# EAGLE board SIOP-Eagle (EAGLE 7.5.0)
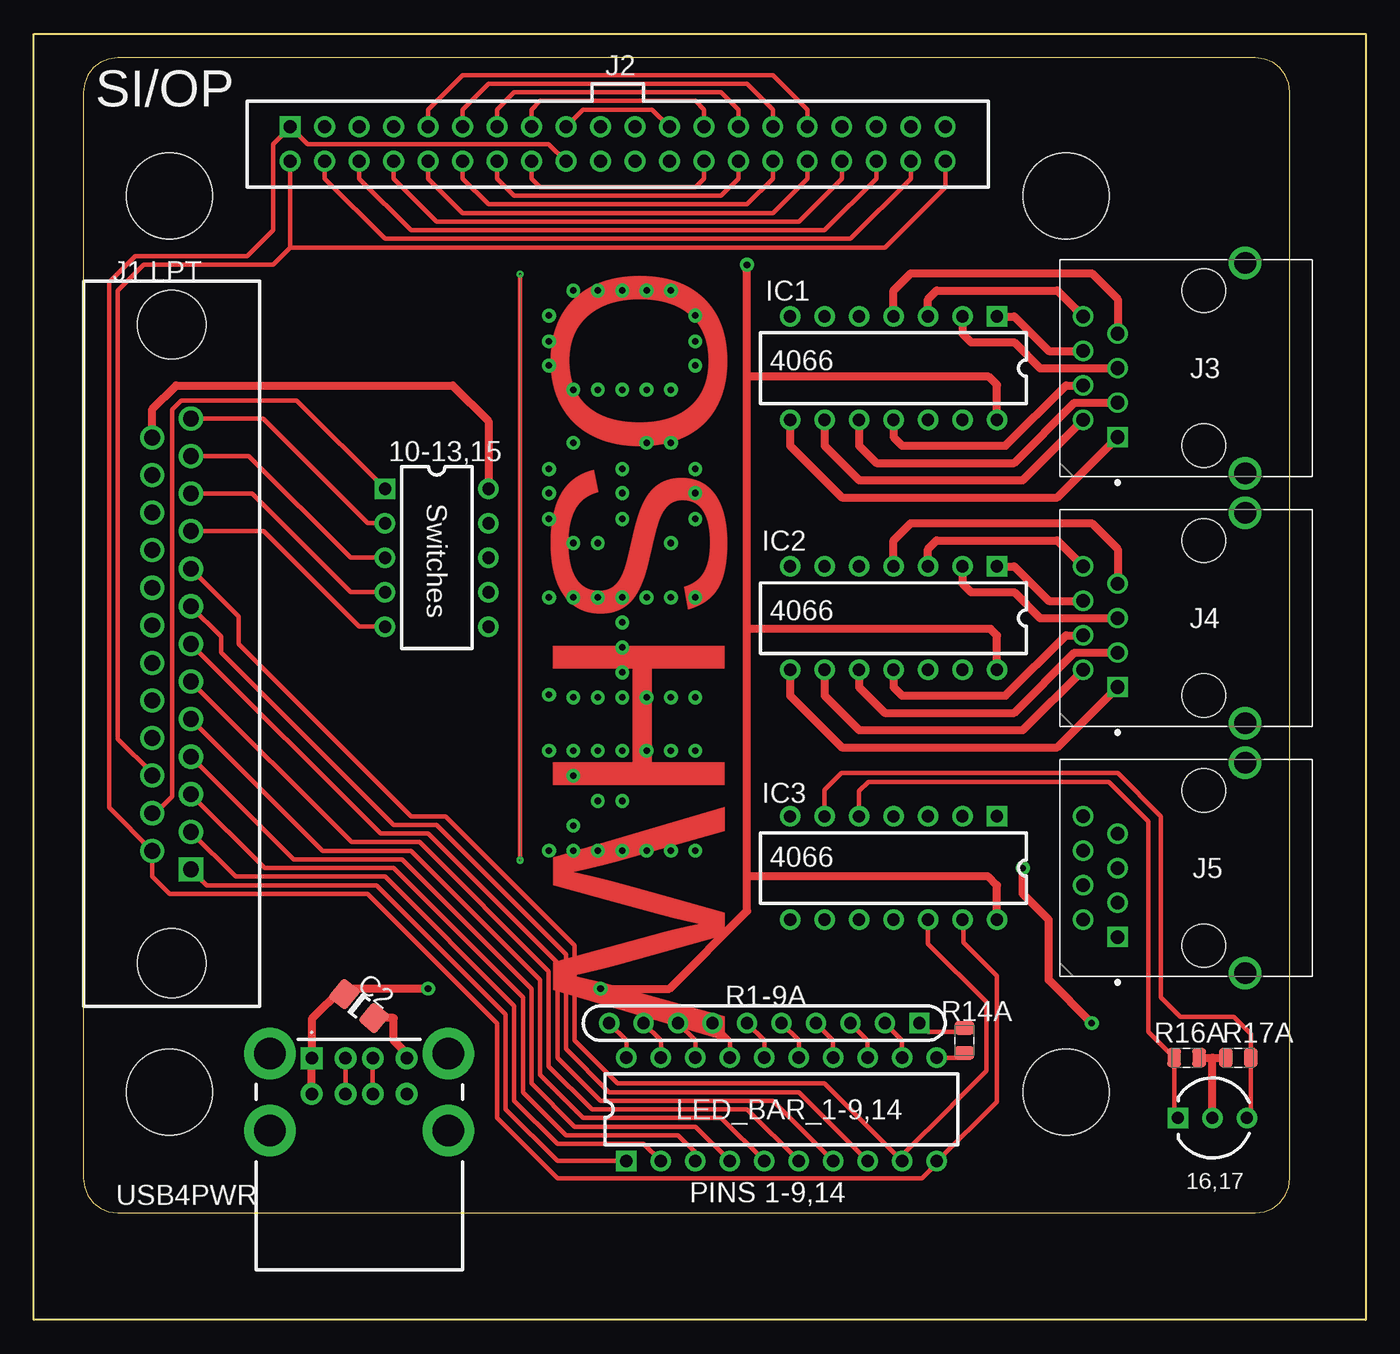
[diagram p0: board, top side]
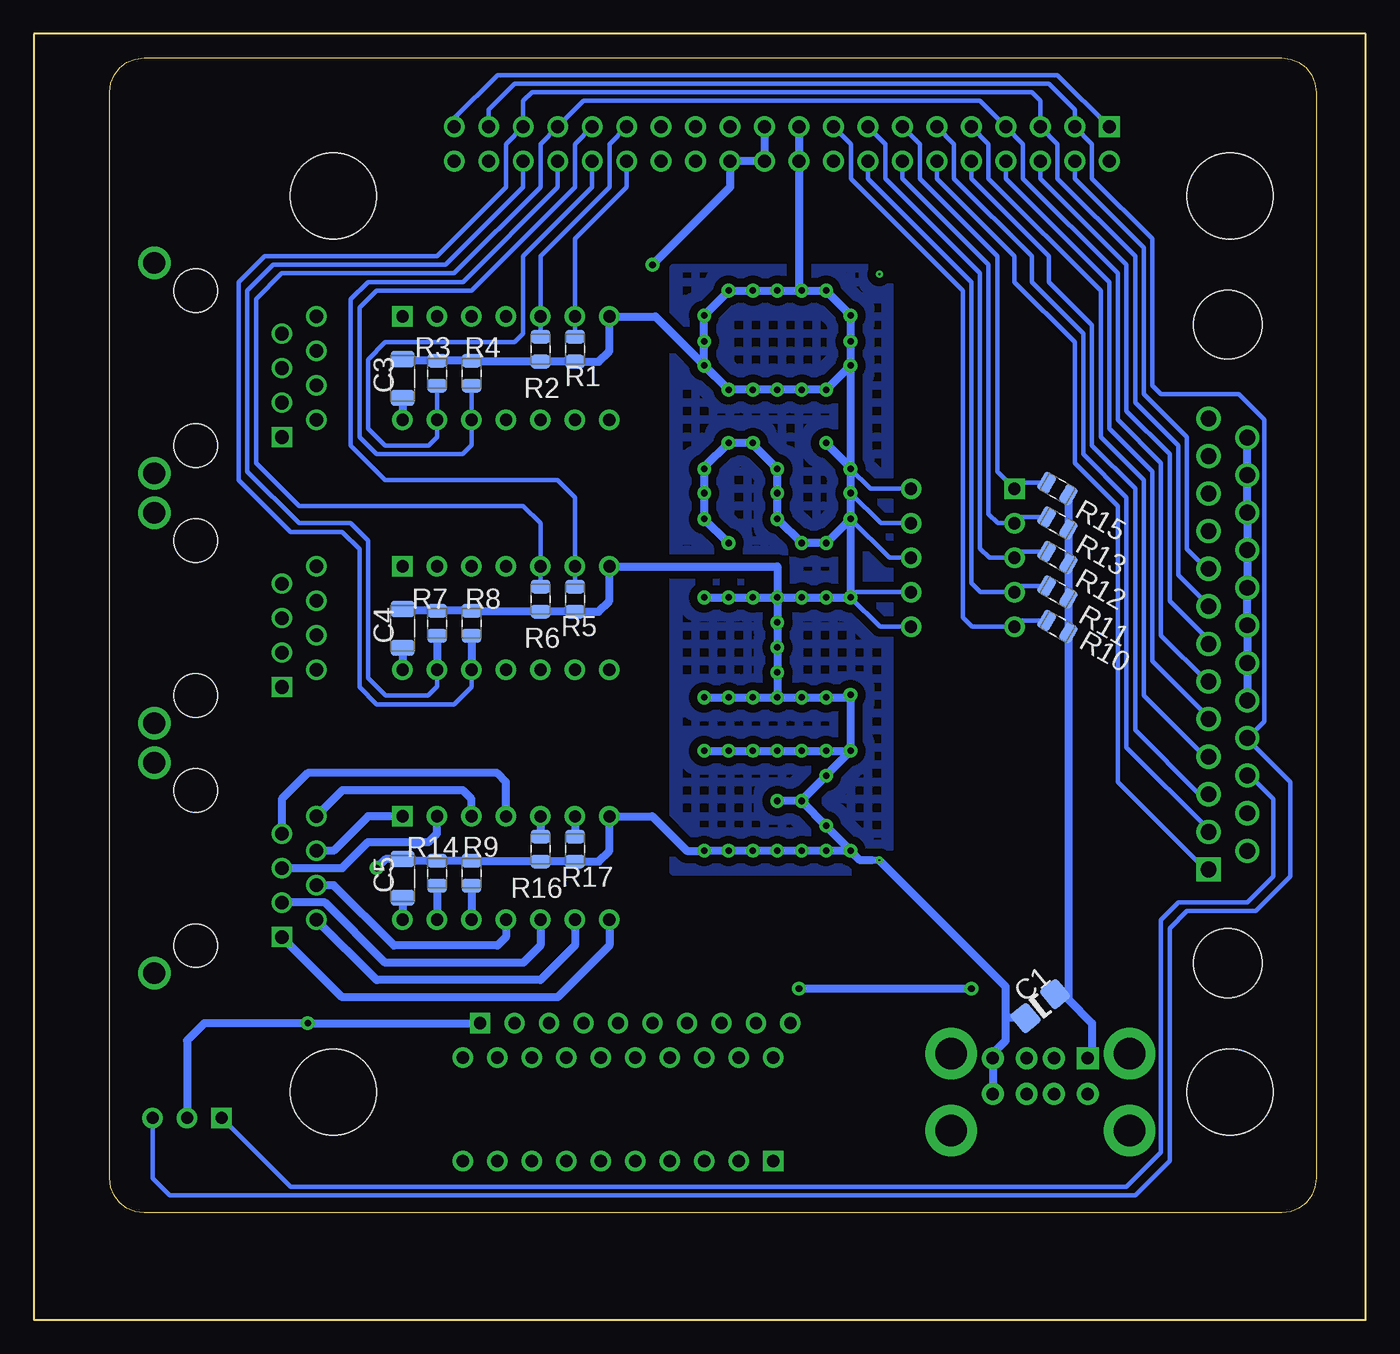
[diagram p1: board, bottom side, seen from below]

Size 98.11 x 94.73 mm. Coordinates in mm from the lower left corner, seen from the top.
Outline: 0,94.73 98.11,94.73 98.11,0 0,0 0,94.73
Copper layers (1*16): Top 0.035mm / dielectric 1.5mm / Bottom 0.035mm
Design rules "default *": minimum track width 10mil, minimum drill 0.61mm, track to track 8mil, track to pad 8mil, pad to pad 8mil, via to via 8mil, smd to smd 8mil, copper to edge 40mil, drill to drill 8mil, minimum pad ring 0mil, minimum via ring 8mil, stop-mask expansion 4mil, vias tented up to drill 40mil, thermal gap 10mil
Net classes: 0 Default: width 0.317 mm, clearance 0.597 mm
Holes 6.35 mm at 9.99,82.81 76.03,82.81 9.99,16.77 76.03,16.77
Milling: 28 lines

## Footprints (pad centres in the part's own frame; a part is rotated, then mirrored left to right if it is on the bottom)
CAP_1206 = smd 1.6 x 1.8: 1 -1.4,0; 2 1.4,0
CAP_1206_C2 = smd 1.6 x 1.8: 1 -1.4,0; 2 1.4,0
CAPC320X160X180L50N_AD1 = smd 1.21 x 1.77: 1 -1.43,0; 2 1.43,0
LED(BI)-5R = drill 0.889 pad 1.5 square: 1 -2.54,0 | drill 0.889 pad 1.5: 2 0,0; 3 2.54,0
DIP-14 = drill 0.9 pad 1.5 square: 1 -3.81,7.62 | drill 0.9 pad 1.5: 2 -3.81,5.08; 3 -3.81,2.54; 4 -3.81,0; 5 -3.81,-2.54; 6 -3.81,-5.08; 7 -3.81,-7.62; 8 3.81,-7.62; 9 3.81,-5.08; 10 3.81,-2.54; 11 3.81,0; 12 3.81,2.54; 13 3.81,5.08; 14 3.81,7.62
DB25F = drill 1.168 pad 1.778 square: 1 16.612,1.422 | drill 1.168 pad 1.778: 2 13.843,1.422; 3 11.074,1.422; 4 8.306,1.422; 5 5.537,1.422; 6 2.769,1.422; 7 0,1.422; 8 -2.769,1.422; 9 -5.537,1.422; 10 -8.306,1.422; 11 -11.074,1.422; 12 -13.843,1.422; 13 -16.612,1.422; 14 15.24,-1.422; 15 12.471,-1.422; 16 9.703,-1.422; 17 6.934,-1.422; 18 4.166,-1.422; 19 1.397,-1.422; 20 -1.372,-1.422; 21 -4.14,-1.422; 22 -6.909,-1.422; 23 -9.677,-1.422; 24 -12.446,-1.422; 25 -15.215,-1.422 | hole 5.08: -23.52,0; 23.52,0
IDC40F = drill 0.965 pad 1.524 square: 1 -24.13,1.27 | drill 0.965 pad 1.524: 2 -24.13,-1.27; 3 -21.59,1.27; 4 -21.59,-1.27; 5 -19.05,1.27; 6 -19.05,-1.27; 7 -16.51,1.27; 8 -16.51,-1.27; 9 -13.97,1.27; 10 -13.97,-1.27; 11 -11.43,1.27; 12 -11.43,-1.27; 13 -8.89,1.27; 14 -8.89,-1.27; 15 -6.35,1.27; 16 -6.35,-1.27; 17 -3.81,1.27; 18 -3.81,-1.27; 19 -1.27,1.27; 20 -1.27,-1.27; 21 1.27,1.27; 22 1.27,-1.27; 23 3.81,1.27; 24 3.81,-1.27; 25 6.35,1.27; 26 6.35,-1.27; 27 8.89,1.27; 28 8.89,-1.27; 29 11.43,1.27; 30 11.43,-1.27; 31 13.97,1.27; 32 13.97,-1.27; 33 16.51,1.27; 34 16.51,-1.27; 35 19.05,1.27; 36 19.05,-1.27; 37 21.59,1.27; 38 21.59,-1.27; 39 24.13,1.27; 40 24.13,-1.27
CKMTW_RJ45-TH_R-RJ45R10P-B000 = drill 1 pad 1.5 square: 1 0,0 | drill 1 pad 1.5: 2 -1.27,-2.54; 3 -2.54,0; 4 -3.81,-2.54; 5 -5.08,0; 6 -6.35,-2.54; 7 -7.62,0; 8 -8.89,-2.54 | drill 1.6 pad 2.4: 9 2.67,9.4; 10 -12.83,9.4 | hole 3.2: -10.795,6.35; 0.635,6.35
DIP-20 = drill 0.9 pad 1.5 square: 1 -3.81,11.43 | drill 0.9 pad 1.5: 2 -3.81,8.89; 3 -3.81,6.35; 4 -3.81,3.81; 5 -3.81,1.27; 6 -3.81,-1.27; 7 -3.81,-3.81; 8 -3.81,-6.35; 9 -3.81,-8.89; 10 -3.81,-11.43; 11 3.81,-11.43; 12 3.81,-8.89; 13 3.81,-6.35; 14 3.81,-3.81; 15 3.81,-1.27; 16 3.81,1.27; 17 3.81,3.81; 18 3.81,6.35; 19 3.81,8.89; 20 3.81,11.43
RESC200X125X60L40N_AD1_R5 = smd 0.99 x 1.42: 1 -0.92,0; 2 0.92,0
SIP-10/26.6x2.4x2.54 = drill 0.9 pad 1.5 square: 1 -11.43,0 | drill 0.9 pad 1.5: 2 -8.89,0; 3 -6.35,0; 4 -3.81,0; 5 -1.27,0; 6 1.27,0; 7 3.81,0; 8 6.35,0; 9 8.89,0; 10 11.43,0
RESC200X125X60L40N_AD1 = smd 0.99 x 1.42: 1 -0.92,0; 2 0.92,0
RESC200X125X60L40N_AD1_R3 = smd 0.99 x 1.42: 1 -0.92,0; 2 0.92,0
RESC200X125X60L40N_AD1_R4 = smd 0.99 x 1.42: 1 -0.92,0; 2 0.92,0
RESC200X125X60L40N_AD1_R10 = smd 0.99 x 1.42: 1 -0.92,0; 2 0.92,0
RESC200X125X60L40N_AD1_R15 = smd 0.99 x 1.42: 1 -0.92,0; 2 0.92,0
RESC200X125X60L40N_AD1_R14A = smd 0.99 x 1.42: 1 -0.92,0; 2 0.92,0
RESC200X125X60L40N_AD1_R16 = smd 0.99 x 1.42: 1 -0.92,0; 2 0.92,0
RESC200X125X60L40N_AD1_R16A = smd 0.99 x 1.42: 1 -0.92,0; 2 0.92,0
RESC200X125X60L40N_AD1_R17 = smd 0.99 x 1.42: 1 -0.92,0; 2 0.92,0
RESC200X125X60L40N_AD1_R17A = smd 0.99 x 1.42: 1 -0.92,0; 2 0.92,0
DIP-10 = drill 0.9 pad 1.5 square: 1 -3.81,5.08 | drill 0.9 pad 1.5: 2 -3.81,2.54; 3 -3.81,0; 4 -3.81,-2.54; 5 -3.81,-5.08; 6 3.81,-5.08; 7 3.81,-2.54; 8 3.81,0; 9 3.81,2.54; 10 3.81,5.08
USB-2.5/4H8D = drill 0.92 pad 1.6 square: 1 -2.49,-3.5 | drill 0.92 pad 1.6: 2 -2.49,-1; 3 -2.49,1; 4 -2.49,3.5; 5 0.13,-3.5; 6 0.13,-1; 7 0.13,1; 8 0.13,3.5 | drill 2.3 pad 3.8: 9 2.84,6.57; 10 2.84,-6.57; 11 -2.84,6.57; 12 -2.84,-6.57

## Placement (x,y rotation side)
C1  CAP_1206  [CAP_1206]  23.96,23.12 39.2 bottom
C2  CAP_1206  [CAP_1206_C2]  23.96,23.12 321 top
C3  EMK316BBJ476ML-T  [CAPC320X160X180L50N_AD1]  70.95,69.35 90 bottom
C4  EMK316BBJ476ML-T  [CAPC320X160X180L50N_AD1]  70.95,50.94 90 bottom
C5  EMK316BBJ476ML-T  [CAPC320X160X180L50N_AD1]  70.95,32.52 90 bottom
D1  5mm Round Bi-Color  [LED(BI)-5R]  86.83,14.87 0 top
IC1  4066  [DIP-14]  63.33,70.11 270 top
IC2  4066  [DIP-14]  63.33,51.7 270 top
IC3  4066  [DIP-14]  63.33,33.28 270 top
J1  LPT  [DB25F]  10.14,49.79 270 top
J2  IDC40F  [IDC40F]  43.01,86.62 0 top
J3  R-RJ45R10P-B000  [CKMTW_RJ45-TH_R-RJ45R10P-B000]  79.84,65.03 270 top
J4  R-RJ45R10P-B000  [CKMTW_RJ45-TH_R-RJ45R10P-B000]  79.84,46.62 270 top
J5  R-RJ45R10P-B000  [CKMTW_RJ45-TH_R-RJ45R10P-B000]  79.84,28.2 270 top
LED_BAR_1-9,14  PINS 1-9,14  [DIP-20]  55.08,15.5 90 top
R1  RS-05K1002FT  [RESC200X125X60L40N_AD1_R5]  58.25,71.51 90 bottom
R1-9A  RES10SIPDT  [SIP-10/26.6x2.4x2.54]  53.81,21.85 180 top
R2  RS-05K1002FT  [RESC200X125X60L40N_AD1]  60.79,71.51 90 bottom
R3  RS-05K1002FT  [RESC200X125X60L40N_AD1_R3]  68.41,69.73 90 bottom
R4  RS-05K1002FT  [RESC200X125X60L40N_AD1_R4]  65.87,69.73 90 bottom
R5  RS-05K1002FT  [RESC200X125X60L40N_AD1_R5]  58.25,53.09 90 bottom
R6  RS-05K1002FT  [RESC200X125X60L40N_AD1]  60.79,53.09 90 bottom
R7  RS-05K1002FT  [RESC200X125X60L40N_AD1_R3]  68.41,51.32 90 bottom
R8  RS-05K1002FT  [RESC200X125X60L40N_AD1_R4]  65.87,51.32 90 bottom
R9  RS-05K1002FT  [RESC200X125X60L40N_AD1_R4]  65.87,32.9 90 bottom
R10  RS-05K1002FT  [RESC200X125X60L40N_AD1_R10]  22.69,51.06 330 bottom
R11  RS-05K1002FT  [RESC200X125X60L40N_AD1_R15]  22.69,53.6 330 bottom
R12  RS-05K1002FT  [RESC200X125X60L40N_AD1_R15]  22.69,56.14 330 bottom
R13  RS-05K1002FT  [RESC200X125X60L40N_AD1_R15]  22.69,58.68 330 bottom
R14  RS-05K1002FT  [RESC200X125X60L40N_AD1_R3]  68.41,32.9 90 bottom
R14A  RS-05K1002FT  [RESC200X125X60L40N_AD1_R14A]  68.54,20.57 90 top
R15  RS-05K1002FT  [RESC200X125X60L40N_AD1_R15]  22.69,61.22 330 bottom
R16  RS-05K1002FT  [RESC200X125X60L40N_AD1_R16]  60.79,34.68 90 bottom
R16A  RS-05K1002FT  [RESC200X125X60L40N_AD1_R16A]  84.92,19.31 0 top
R17  RS-05K1002FT  [RESC200X125X60L40N_AD1_R17]  58.25,34.68 90 bottom
R17A  RS-05K1002FT  [RESC200X125X60L40N_AD1_R17A]  88.73,19.31 0 top
Switches  10-13,15  [DIP-10]  29.68,56.14 0 top
USB4PWR  USB-2.5/4H8D  [USB-2.5/4H8D]  23.96,16.77 270 top

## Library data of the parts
C1 C2 = common; UNIQUE_NAME: CAP_1206
C3-C5 = common; MANUFACTURER: Taiyo Yuden; PART_NUMBER_(LCSC): C385907; UNIQUE_NAME: TAIYO_MK316(1206)
D1 = common; DATASHEET: http://datasheets.diptrace.com/sensors_led/WP59EGC.pdf; MANUFACTURER: Kingbright; UNTITLED: 16,17
IC1-IC3 J1 J2 LED_BAR_1-9,14 R1-9A Switches USB4PWR = common
J3-J5 = common; DATASHEET: http://datasheets.diptrace.com/ckmtw/R-RJ45R10P-B000.pdf; MANUFACTURER: Ckmtw(Shenzhen Cankemeng); PART_NUMBER_(LCSC): C386758; UNIQUE_NAME: CKMTW_RJ45-TH_R-RJ45R10P-B000
R1-R14 R14A R15 R16 R16A R17 R17A = common; DATASHEET: http://datasheets.diptrace.com/fh/RS-03K1000FT_and_series.pdf; MANUFACTURER: FH(Guangdong Fenghua Advanced Tech); PART_NUMBER_(LCSC): C115309; UNIQUE_NAME: FH_0805_H0.5

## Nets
Net_0: C1.1 C2.2 C3.2 C4.2 C5.2 D1.2 IC1.7 IC2.7 IC3.7 J1.18 J1.19 J1.20 J1.21 J1.22 J1.23 J1.24 J1.25 J2.19 J2.20 R1-9A.1 R1.1 R2.1 R3.2 R4.2 R5.1 R6.1 R7.2 R8.2 R9.2 R14.2 R14A.2 R16.1 R16A.2 R17.1 R17A.1 Switches.6 Switches.7 Switches.8 Switches.9 Switches.10 USB4PWR.4 USB4PWR.8
Net_2: IC1.3 J3.8
Net_3: IC1.4 J3.7
Net_4: IC1.2 J3.5
Net_5: IC1.11 J3.4
Net_6: IC1.9 J3.2
Net_7: IC1.8 J3.1
Net_8: D1.1 IC3.5 J1.16 J2.2 J2.40 R16.2 R16A.1
Net_9: IC1.10 J3.3
Net_10: IC1.12 J1.4 J2.9 J2.31 LED_BAR_1-9,14.4 R4.1
Net_11: IC2.12 J1.8 J2.5 J2.35 LED_BAR_1-9,14.8 R8.1
Net_12: IC2.5 J1.6 J2.7 J2.33 LED_BAR_1-9,14.6 R6.2
Net_14: IC2.13 J1.7 J2.6 J2.36 LED_BAR_1-9,14.7 R7.1
Net_15: D1.3 IC3.6 J1.17 J2.3 J2.37 R17.2 R17A.2
Net_16: IC2.1 J4.6
Net_17: IC1.6 J1.1 J2.12 J2.30 LED_BAR_1-9,14.1 R1.2
Net_18: IC1.5 J1.2 J2.11 J2.29 LED_BAR_1-9,14.2 R2.2
Net_19: IC1.13 J1.3 J2.10 J2.32 LED_BAR_1-9,14.3 R3.1
Net_20: J1.15 J2.13 J2.27 R15.1 Switches.1
Net_21: IC2.6 J1.5 J2.8 J2.34 LED_BAR_1-9,14.5 R5.2
Net_22: LED_BAR_1-9,14.20 R1-9A.10
Net_24: LED_BAR_1-9,14.19 R1-9A.9
Net_25: IC3.12 J1.9 J2.4 J2.38 LED_BAR_1-9,14.9 R9.1
Net_26: LED_BAR_1-9,14.18 R1-9A.8
Net_27: IC3.13 J1.14 J2.1 J2.18 J2.39 LED_BAR_1-9,14.10 R14.1
Net_28: C1.2 C2.1 C3.1 C4.1 C5.1 IC1.14 IC2.14 IC3.14 J2.21 J2.22 J2.24 R10.2 R11.2 R12.2 R13.2 R15.2 USB4PWR.1 USB4PWR.5
Net_29: IC1.1 J3.6
Net_30: LED_BAR_1-9,14.17 R1-9A.7
Net_31: LED_BAR_1-9,14.16 R1-9A.6
Net_32: LED_BAR_1-9,14.14 R1-9A.4
Net_33: LED_BAR_1-9,14.13 R1-9A.3
Net_34: LED_BAR_1-9,14.12 R1-9A.2
Net_35: USB4PWR.2 USB4PWR.6
Net_36: USB4PWR.3 USB4PWR.7
Net_37: LED_BAR_1-9,14.11 R14A.1
Net_43: IC2.3 J4.8
Net_44: IC2.4 J4.7
Net_45: IC2.2 J4.5
Net_46: IC2.11 J4.4
Net_47: IC2.9 J4.2
Net_48: J1.10 J2.17 J2.23 R10.1 Switches.5
Net_49: IC2.8 J4.1
Net_50: IC2.10 J4.3
Net_51: J1.12 J2.15 J2.25 R12.1 Switches.3
Net_56: LED_BAR_1-9,14.15 R1-9A.5
Net_57: IC3.1 J5.6
Net_58: IC3.3 J5.8
Net_59: IC3.4 J5.7
Net_60: IC3.2 J5.5
Net_61: IC3.11 J5.4
Net_62: IC3.9 J5.2
Net_63: IC3.8 J5.1
Net_64: IC3.10 J5.3
Net_69: J1.13 J2.14 J2.28 R13.1 Switches.2
Net_70: J1.11 J2.16 J2.26 R11.1 Switches.4

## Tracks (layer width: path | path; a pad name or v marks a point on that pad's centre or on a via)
N$1
  pour Bottom (isolate 0.33, no thermals, hatched): 35.12,77.48 51,77.48 51,33.03 35.12,33.03
Net_0  (via drill 0.13 pad 0.51, 0.49 pad 1.02)
  Top 0.315: v35.82,77.03 v35.82,33.85
  Top 0.318: R14A.2 68.54,21.22 65.87,21.22 R1-9A.1
  Top 0.597: J1.25 8.72,67.09 10.47,68.84 30.85,68.84 33.49,66.21 Switches.10 | USB4PWR.4 27.46,19.62 26.5,20.58 26.5,22.24 C2.2 | R16A.2 86.83,19.31 | 86.83,19.31 | 86.83,19.31 R17A.1 | D1.2 86.83,19.31 | v77.94,21.85 | v77.94,21.85 74.76,25.03 74.76,29.47 72.86,31.38 v72.86,33.28
  Bottom 0.318: Switches.10 36.48,61.22 v37.94,62.68 | Switches.9 35.72,58.68 v37.94,60.91 | Switches.8 35.08,56.14 v37.94,59 | Switches.7 37.56,53.6 v37.94,53.22 35.78,51.06 Switches.6
  Bottom 0.508: v35.82,33.85 36.37,33.85
  Bottom 0.597: J1.18 J1.19 J1.20 J1.21 J1.22 J1.23 J1.24 J1.25 | 36.37,33.85 37.24,33.85 v37.94,34.55 | R2.1 R1.1 56.5,70.59 55.71,71.38 IC1.7 52.33,73.92 v46.93,68.52 | R2.1 | R2.1 65.81,70.59 R4.2 R3.2 | R3.2 | R3.2 70.82,70.65 C3.2 | v41.54,68.52 v39.75,68.52 39.72,68.52 v37.94,70.3 | v41.54,68.52 | v41.54,68.52 v43.34,68.52 | v43.34,68.52 | v43.34,68.52 v45.14,68.52 | v45.14,68.52 | v45.14,68.52 v46.93,68.52 | v46.93,68.52 | v46.93,68.52 46.95,68.52 v48.73,70.3 v48.73,72.08 v48.73,73.99 46.93,75.78 v46.93,75.83 v45.14,75.83 | v45.14,75.83 | v45.14,75.83 v43.34,75.83 | v43.34,75.83 | v43.34,75.83 v41.54,75.83 | v41.54,75.83 | v41.54,75.83 v39.75,75.83 | v39.75,75.83 | v37.94,70.3 v37.94,72.08 v37.94,73.99 37.94,74.02 v39.75,75.83 | v37.94,70.3 v37.94,62.68 | v39.75,64.6 37.94,62.8 v37.94,62.68 | v37.94,62.68 v37.94,60.91 v37.94,59 | v37.94,59 39.72,57.22 v39.75,57.22 v41.54,57.22 | v41.54,57.22 | v41.54,57.22 43.31,59 v43.34,59 v43.34,60.91 v43.34,62.68 45.14,64.48 v45.14,64.6 v46.93,64.6 | v46.93,64.6 | v46.93,64.6 48.73,62.81 v48.73,62.68 v48.73,60.91 v48.73,59 46.95,57.22 v46.93,57.22 | v37.94,59 v37.94,53.22 | v48.73,53.22 v46.93,53.22 | v46.93,53.22 | v46.93,53.22 v45.14,53.22 | v45.14,53.22 | v45.14,53.22 v43.34,53.22 | v43.34,53.22 | v43.34,53.22 v41.54,53.22 | v41.54,53.22 | v41.54,53.22 v39.75,53.22 | v39.75,53.22 | v39.75,53.22 v37.94,53.22 | v37.94,53.22 | v43.34,53.22 v43.34,51.38 v43.34,49.54 | v43.34,49.54 v43.34,47.7 v43.34,45.85 | v48.73,45.85 v46.93,45.85 | v46.93,45.85 | v46.93,45.85 v45.14,45.85 | v45.14,45.85 | v45.14,45.85 v43.34,45.85 | v43.34,45.85 | v43.34,45.85 v41.54,45.85 | v41.54,45.85 | v41.54,45.85 v39.75,45.85 | v39.75,45.85
  Bottom 0.597: v39.75,45.85 37.94,45.85 v37.94,46.05 v37.94,41.92 | v48.73,41.92 v46.93,41.92 | v46.93,41.92 | v46.93,41.92 v45.14,41.92 | v45.14,41.92 | v45.14,41.92 v43.34,41.92 | v43.34,41.92 | v43.34,41.92 v41.54,41.92 | v41.54,41.92 | v41.54,41.92 v39.75,41.92 | v39.75,41.92 | v39.75,41.92 v37.94,41.92 | v37.94,41.92 | v37.94,41.92 39.75,40.12 v39.75,40.08 41.54,38.29 v41.54,38.22 | v41.54,38.22 v43.34,38.22 | v43.34,38.22 | v41.54,38.22 41.54,38.19 v39.75,36.39 37.94,34.59 v37.94,34.55 | v37.94,34.55 v39.75,34.55 | v39.75,34.55 | v39.75,34.55 v41.54,34.55 | v41.54,34.55 | v41.54,34.55 v43.34,34.55 | v43.34,34.55 | v43.34,34.55 v45.14,34.55 | v45.14,34.55 | v45.14,34.55 v46.93,34.55 | v46.93,34.55 | v46.93,34.55 v48.73,34.55 | v48.73,34.55 | R6.1 R5.1 56.5,52.17 55.71,52.97 IC2.7 43.34,55.51 v43.34,49.54 | R6.1 | R6.1 65.81,52.17 R8.2 R7.2 | R7.2 | R7.2 70.82,52.24 C4.2 | R16.1 R17.1 56.5,33.76 55.71,34.55 IC3.7 52.54,37.09 50,34.55 v48.73,34.55 | R16.1 | R16.1 65.81,33.76 R9.2 R14.2 | R14.2 | R14.2 70.82,33.82 C5.2 72.19,33.95 v72.86,33.28 | J2.19 J2.20 41.74,76.03 v41.54,75.83 | USB4PWR.8 USB4PWR.4 27.46,19.62 26.5,20.58 26.5,22.24 | 26.5,22.24 26.5,24.53 v35.82,33.85 | R1-9A.1 v77.94,21.85 85.56,21.85 86.83,20.58 D1.2 | C2.2 26.5,22.24
Net_2
  Top 0.597: IC1.3 65.87,75.19 66.51,75.83 75.4,75.83 J3.8
Net_3
  Top 0.597: IC1.4 63.33,75.83 64.6,77.1 77.94,77.1 79.84,75.19 J3.7
Net_4
  Top 0.597: IC1.2 68.41,72.65 69.05,72.02 72.22,72.02 74.13,70.11 J3.5
Net_5
  Top 0.597: IC1.11 63.33,65.03 63.97,64.4 71.59,64.4 76.03,68.84 J3.4
Net_6
  Top 0.597: IC1.9 58.25,64.4 60.79,61.86 72.86,61.86 J3.2
Net_7
  Top 0.597: IC1.8 55.71,64.4 59.52,60.59 75.4,60.59 J3.1
Net_8
  Top 0.318: D1.1 84,15.15 R16A.1 82.11,21.2 82.11,36.73 79.21,39.63 61.47,39.63 60.79,38.96 IC3.5 | J1.16 8.72,40.27 6.18,42.81 6.18,75.83 8.09,77.73 17.61,77.73 18.88,79 | 18.88,79 J2.2 18.88,79 | 18.88,79 62.7,79 67.14,83.45 J2.40
  Bottom 0.318: J1.16 8.54,40.09 6.82,38.36 6.82,32.65 8.72,30.74 13.8,30.74 15.07,29.47 15.07,12.33 17.61,9.79 79.21,9.79 D1.1
  Bottom 0.597: IC3.5 R16.2 | R16.2
Net_9
  Top 0.597: IC1.10 60.79,64.4 62.06,63.13 72.22,63.13 76.67,67.57 J3.3
Net_10
  Top 0.318: J2.9 29.04,89.16 31.58,91.7 54.44,91.7 56.98,89.16 J2.31 | LED_BAR_1-9,14.4 48.73,14.23 39.84,14.23 36.66,17.41 36.66,24.39 27.14,33.92 19.14,33.92 J1.4 | J2.31 | J2.31
  Bottom 0.318: J1.4 11.84,41.49 16.34,45.98 16.34,61.86 19.52,65.03 19.52,75.83 27.77,84.08 27.77,86.62 J2.9 | J2.31 58.25,86.62 58.25,83.45 65.87,75.83 72.86,75.83 74.13,74.56 74.13,65.03 72.86,63.76 66.55,63.76 65.87,64.44 IC1.12 R4.1 | R4.1
Net_11
  Top 0.318: LED_BAR_1-9,14.8 56.35,16.77 42.38,16.77 39.2,19.95 39.2,26.93 29.68,36.46 26.5,36.46 13.8,49.16 13.8,50.33 J1.8
  Bottom 0.318: J1.8 11.57,52.64 13.8,54.87 13.8,64.4 16.98,67.57 16.98,78.37 22.69,84.08 22.69,86.62 J2.5 23.96,89.8 24.6,90.43 61.43,90.43 62.06,89.8 J2.35 63.33,86.62 63.33,83.45 68.41,78.37 81.11,78.37 83.02,76.46 83.02,61.86 79.21,58.05 75.4,58.05 74.13,56.78 74.13,46.62 72.86,45.35 67.14,45.35 65.87,46.62 IC2.12
  Bottom 0.597: R8.1 IC2.12 | IC2.12
Net_12
  Top 0.318: LED_BAR_1-9,14.6 | LED_BAR_1-9,14.6 52.54,15.5 41.11,15.5 37.93,18.68 37.93,25.66 28.41,35.19 23.4,35.19 J1.6
  Bottom 0.318: J1.6 11.67,47.02 15.07,50.43 15.07,63.13 18.25,66.3 18.25,77.1 25.23,84.08 25.23,86.62 J2.7 28.41,89.8 57.62,89.8 J2.33 60.79,86.62 60.79,83.45 67.14,77.1 79.84,77.1 81.75,75.19 81.75,63.13 78.57,59.95 62.06,59.95 60.79,58.68 IC2.5 R6.2 | R6.2
Net_14
  Top 0.318: J2.6 23.96,84.08 27.77,80.27 58.25,80.27 62.06,84.08 J2.36 | LED_BAR_1-9,14.7 54.44,16.14 41.74,16.14 38.57,19.31 38.57,26.3 29.04,35.82 25.54,35.82 J1.7
  Bottom 0.318: J1.7 11.57,50.1 14.44,52.97 14.44,63.76 17.61,66.94 17.61,77.73 23.96,84.08 J2.6 | J2.36 62.06,83.45 67.78,77.73 80.48,77.73 82.38,75.83 82.38,62.49 78.57,58.68 74.76,58.68 73.49,57.41 73.49,47.29 72.18,45.98 69.09,45.98 68.41,46.66 IC2.13
  Bottom 0.597: R7.1 IC2.13 | IC2.13
Net_15
  Top 0.318: D1.3 89.65,15.15 R17A.2 89.65,21.06 88.39,22.32 84.45,22.32 83.02,23.76 83.02,37.09 79.84,40.27 59.48,40.27 58.25,39.04 IC3.6
  Bottom 0.318: J2.37 64.6,89.16 62.7,91.07 23.33,91.07 21.42,89.16 J2.3 20.15,86.62 20.15,84.08 15.71,79.64 15.71,68.84 15.07,68.21 9.36,68.21 7.45,66.3 7.45,44.08 8.67,42.86 J1.17 8.72,42.81 5.55,39.63 5.55,32.65 8.09,30.11 13.17,30.11 14.44,28.84 14.44,11.69 16.98,9.15 88.1,9.15 89.37,10.42 D1.3
  Bottom 0.597: IC3.6 R17.2 | R17.2
Net_16
  Top 0.597: IC2.1 72.22,55.51 74.76,52.97 J4.6
Net_17
  Top 0.318: J2.12 31.58,84.08 33.49,82.18 52.54,82.18 54.44,84.08 J2.30 | LED_BAR_1-9,14.1 38.57,11.69 34.76,15.5 34.76,22.49 25.23,32.01 12.73,32.01 J1.1
  Bottom 0.318: J1.1 11.79,33.18 18.25,39.63 18.25,59.95 21.42,63.13 21.42,72.02 25.87,76.46 25.87,78.37 31.58,84.08 J2.12 | R1.2 IC1.6 | IC1.6 | IC1.6 58.25,79.64 54.44,83.45 J2.30
Net_18
  Top 0.318: J2.11 31.58,89.16 33.49,91.07 52.54,91.07 54.44,89.16 J2.29 | LED_BAR_1-9,14.2 44.92,12.96 38.57,12.96 35.39,16.14 35.39,23.12 25.87,32.65 14.87,32.65 J1.2
  Bottom 0.318: J1.2 11.57,36.13 17.61,42.17 17.61,60.59 20.79,63.76 20.79,72.65 24.6,76.46 24.6,78.37 30.31,84.08 30.31,86.62 J2.11 | R2.2 IC1.5 | IC1.5 | IC1.5 60.79,78.37 55.71,83.45 55.71,86.62 J2.29
Net_19
  Top 0.318: J2.10 29.04,84.08 31.58,81.54 54.44,81.54 56.98,84.08 J2.32 | LED_BAR_1-9,14.3 48.73,12.33 47.46,13.6 39.2,13.6 36.03,16.77 36.03,23.76 26.5,33.28 17,33.28 J1.3
  Bottom 0.318: J1.3 12.25,38.72 16.98,43.44 16.98,61.22 20.15,64.4 20.15,73.29 23.33,76.46 23.33,78.37 29.04,84.08 J2.10 | J2.32 56.98,83.45 62.06,78.37 62.06,72.65 62.7,72.02 72.22,72.02 73.49,70.75 73.49,65.67 72.22,64.4 69.05,64.4 68.41,65.03 IC1.13 R3.1 | R3.1
Net_20
  Top 0.318: J2.13 34.12,89.16 35.39,90.43 50.63,90.43 51.9,89.16 J2.27 | J1.15 8.95,37.32 10.18,38.55 10.18,67.05 10.85,67.72 19.37,67.72 Switches.1
  Bottom 0.318: R15.1 25.41,61.68 Switches.1 27.14,62.49 27.14,78.37 32.85,84.08 32.85,86.62 J2.13
Net_21
  Top 0.318: J2.8 26.5,84.08 29.68,80.91 56.35,80.91 59.52,84.08 J2.34 | LED_BAR_1-9,14.5 | LED_BAR_1-9,14.5 50.63,14.87 40.47,14.87 37.3,18.04 37.3,25.03 27.77,34.55 21.27,34.55 J1.5
  Bottom 0.318: J1.5 11.57,44.38 15.71,48.52 15.71,62.49 18.88,65.67 18.88,76.46 26.5,84.08 J2.8 | R5.2 IC2.6 58.25,60.59 59.52,61.86 72.22,61.86 74.76,64.4 74.76,75.19 73.49,76.46 66.51,76.46 59.52,83.45 J2.34 | R5.2
Net_22
  Top 0.318: LED_BAR_1-9,14.20 43.65,20.58 R1-9A.10
Net_24
  Top 0.318: LED_BAR_1-9,14.19 46.19,20.58 R1-9A.9
Net_25
  Top 0.318: J2.4 21.42,84.08 25.87,79.64 60.16,79.64 64.6,84.08 J2.38 | LED_BAR_1-9,14.9 | LED_BAR_1-9,14.9 58.25,17.41 43.01,17.41 39.84,20.58 39.84,27.57 30.31,37.09 27.77,37.09 15.07,49.79 15.07,51.82 J1.9 | LED_BAR_1-9,14.9 63.97,12.1 67.63,15.77 67.63,15.8 70.16,18.33 70.16,23.41 65.87,27.7 IC3.12
  Bottom 0.318: J1.9 11.72,55.33 13.17,56.78 13.17,65.03 16.34,68.21 16.34,79 21.42,84.08 J2.4
  Bottom 0.597: R9.1 IC3.12 | IC3.12
Net_26
  Top 0.318: LED_BAR_1-9,14.18 48.73,20.58 R1-9A.8
Net_27
  Top 0.318: IC3.13 68.48,29.47 68.48,27.8 70.95,25.33 70.95,16.06 66.58,11.69 LED_BAR_1-9,14.10 66.51,11.5 65.43,10.42 38.57,10.42 34.12,14.87 34.12,21.85 24.6,31.38 9.99,31.38 8.72,32.65 J1.14 5.55,37.73 5.55,76.46 7.45,78.37 15.71,78.37 17.61,80.27 17.61,86.62 J2.1 20.15,86.62 37.93,86.62 J2.18
  Bottom 0.318: J2.1 22.69,91.7 63.97,91.7 67.14,88.53 J2.39
  Bottom 0.597: R14.1 IC3.13 | IC3.13
Net_28  (via drill 0.49 pad 1.02)
  Top 0.597: IC3.14 70.95,32.01 70.32,32.65 52.54,32.65 | 52.54,32.65 52.54,50.9 | 52.54,50.9 52.54,69.48 | 52.54,69.48 v52.54,77.73 | IC2.14 70.95,50.43 70.48,50.9 52.54,50.9 | IC1.14 70.95,68.88 70.36,69.48 52.54,69.48 | USB4PWR.5 USB4PWR.1 20.46,22.16 22.69,24.39 | v29.04,24.39 22.69,24.39 | C2.1 22.69,24.39 | v41.74,24.39 | v41.74,24.39 46.82,24.39 52.54,30.11 52.54,32.65
  Bottom 0.597: C3.1 IC1.14 | C4.1 IC2.14 | IC2.14 | C5.1 IC3.14 | IC3.14 | J2.21 J2.22 J2.24 | J2.24 | J2.24 46.82,83.45 v52.54,77.73 | v29.04,24.39 v41.74,24.39 | v41.74,24.39 | R15.2 R13.2 | R13.2 | R13.2 R12.2 | R12.2 | R12.2 R11.2 R10.2 21.89,23.6 | 21.89,23.6 20.15,21.85 20.15,19.57 USB4PWR.1 | 21.89,23.6 22.04,23.74 22.61,23.74 C2.1
Net_29
  Top 0.597: IC1.1 72.22,73.92 74.76,71.38 J3.6
Net_30
  Top 0.318: LED_BAR_1-9,14.17 51.27,20.58 R1-9A.7
Net_31
  Top 0.318: LED_BAR_1-9,14.16 53.81,20.58 R1-9A.6
Net_32
  Top 0.318: LED_BAR_1-9,14.14 58.89,20.58 R1-9A.4
Net_33
  Top 0.318: LED_BAR_1-9,14.13 61.43,20.58 R1-9A.3
Net_34
  Top 0.318: LED_BAR_1-9,14.12 63.97,20.58 R1-9A.2
Net_35
  Top 0.318: USB4PWR.2 USB4PWR.6 | USB4PWR.6
Net_36
  Top 0.318: USB4PWR.3 USB4PWR.7 | USB4PWR.7
Net_37
  Top 0.318: LED_BAR_1-9,14.11 68.54,19.31 R14A.1
Net_43
  Top 0.597: IC2.3 65.87,56.78 66.51,57.41 75.4,57.41 J4.8
Net_44
  Top 0.597: IC2.4 63.33,57.41 64.6,58.68 77.94,58.68 79.84,56.78 J4.7
Net_45
  Top 0.597: IC2.2 68.41,54.24 69.05,53.6 72.22,53.6 74.13,51.7 J4.5
Net_46
  Top 0.597: IC2.11 63.33,46.62 63.97,45.98 71.59,45.98 76.03,50.43 J4.4
Net_47
  Top 0.597: IC2.9 58.25,45.98 60.79,43.44 72.86,43.44 J4.2
Net_48
  Top 0.318: J2.17 40.47,89.16 45.55,89.16 J2.23 | J1.10 16.93,58.1 23.96,51.06 Switches.5
  Bottom 0.318: J2.17 37.93,86.62 37.93,84.08 29.68,75.83 29.68,51.74 29,51.06 Switches.5 25.41,51.52 R10.1
Net_49
  Top 0.597: IC2.8 55.71,45.98 59.52,42.17 75.39,42.17 J4.1
Net_50
  Top 0.597: IC2.10 60.79,46.62 62.7,44.71 72.22,44.71 76.67,49.16 J4.3
Net_51
  Top 0.318: J2.15 36.66,89.16 37.3,89.8 48.73,89.8 49.36,89.16 J2.25 | J1.12 15.83,63.64 23.33,56.14 Switches.3
  Bottom 0.318: J2.15 35.39,86.62 35.39,84.08 28.41,77.1 28.41,56.82 27.73,56.14 Switches.3 25.41,56.6 R12.1
Net_56
  Top 0.318: LED_BAR_1-9,14.15 56.35,20.58 R1-9A.5
Net_57
  Bottom 0.597: IC3.1 73.49,37.09 76.03,34.55 J5.6
Net_58
  Bottom 0.597: IC3.3 65.87,38.36 66.51,39 75.4,39 J5.8
Net_59
  Bottom 0.597: IC3.4 63.33,39.63 63.97,40.27 77.94,40.27 79.84,38.36 J5.7
Net_60
  Bottom 0.597: J5.5 75.4,33.28 73.49,35.19 69.05,35.19 68.41,35.82 IC3.2
Net_61
  Bottom 0.597: IC3.11 63.33,28.2 63.97,27.57 71.58,27.57 76.03,32.01 J5.4
Net_62
  Bottom 0.597: IC3.9 58.25,27.57 60.79,25.03 72.86,25.03 J5.2
Net_63
  Bottom 0.597: IC3.8 55.71,27.57 59.52,23.76 75.4,23.76 J5.1
Net_64
  Bottom 0.597: IC3.10 60.79,27.57 62.06,26.3 72.22,26.3 76.67,30.74 J5.3
Net_69
  Top 0.318: J2.14 34.12,84.08 35.39,82.81 50.63,82.81 51.9,84.08 J2.28 | J1.13 16.87,66.41 24.6,58.68 Switches.2
  Bottom 0.318: J2.14 34.12,84.08 27.77,77.73 27.77,59.36 27.1,58.68 Switches.2 25.41,59.14 R13.1
Net_70
  Top 0.318: J2.16 36.66,84.08 37.3,83.45 48.73,83.45 49.36,84.08 J2.26 | J1.11 16.06,60.87 23.33,53.6 Switches.4
  Bottom 0.318: J2.16 36.66,84.08 29.04,76.46 29.04,54.28 28.37,53.6 Switches.4 25.41,54.06 R11.1

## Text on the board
Top: OSHW
tPlace: J2 | SI/OP | J1 | LPT | IC1 | 4066 | J3 | 10-13,15 | Switches | IC2 | 4066 | J4 | IC3 | 4066 | J5 | C2 | R1-9A | R14A | R16A | R17A | LED_BAR_1-9,14 | USB4PWR | PINS 1-9,14
bPlace: R1 | R4 | R3 | C3 | R2 | R15 | R13 | R12 | R8 | R7 | R11 | R5 | R10 | R6 | C4 | R17 | R9 | R14 | C5 | R16 | C1
bDocu: remote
